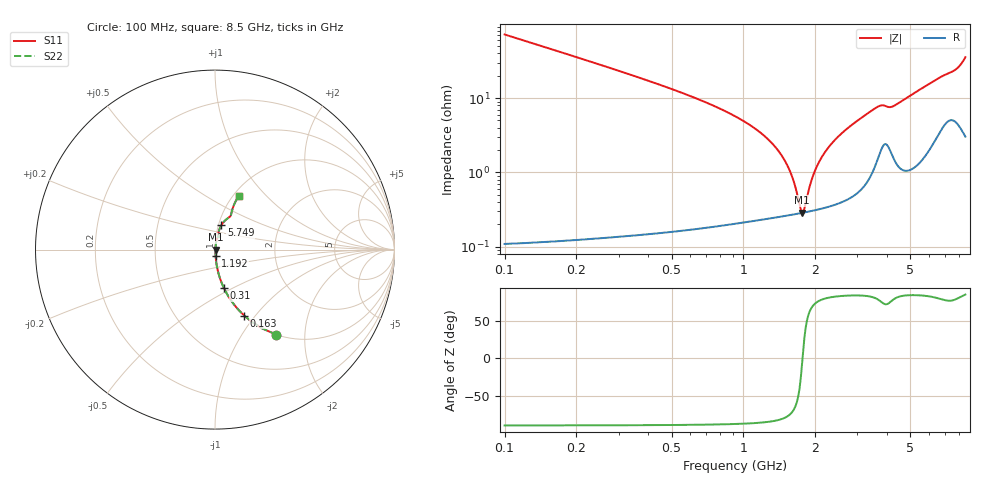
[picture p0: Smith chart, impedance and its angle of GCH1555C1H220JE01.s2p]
!Murata Part Number: GCH1555C1H220JE01
!These Parameters are Measured in Series Mode Connection
!Data Generated on Jun 19, 2026
!  o--ll--o
!Port1  Port2
!  o------o
!Operation Temp=25[degC], DC Bias Voltage=0[V]
!Freq. Start=100[MHz] Stop=9[GHz] 401[Steps]
# Hz S RI R 50
!Freq.(Hz) S11(Real) S11(Imag) S21(Real) S21(Imag) S12(Real) S12(Imag) S22(Real) S22(Imag)
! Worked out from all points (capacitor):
!   401 points, 100 MHz to 8.5 GHz, reference 50 ohm
!   read as one part in series: C = 22 pF near 142 MHz
!   lowest |Z| = 287 mohm at 1.759 GHz (marker M1)
!   series resonance near 1.768 GHz, so ESL is about 370 pH
!   S11 on the Smith chart (normalised r, x): 100 MHz: 1.00, -1.44; 163 MHz: 1.00, -0.88; 310 MHz: 1.00, -0.45; 1.192 GHz: 1.00, -0.07; 5.749 GHz: 1.03, +0.29; 8.5 GHz: 1.06, +0.71
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1e8  0.3422 -0.4737  0.6578 0.4737  0.6578 0.4737  0.3422 -0.4737
1.63e8  0.1628 -0.3678  0.8372 0.3678  0.8372 0.3678  0.1628 -0.3678
3.1e8  0.0497 -0.2144  0.9503 0.2144  0.9503 0.2144  0.0497 -0.2144
6.25e8  0.0118 -0.0998  0.9882 0.0998  0.9882 0.0998  0.0118 -0.0998
1.192e9  0.00339 -0.033  0.9966 0.033  0.9966 0.033  0.00339 -0.033
1.381e9  0.00289 -0.0204  0.9971 0.0204  0.9971 0.0204  0.00289 -0.0204
1.507e9  0.00277 -0.0132  0.9972 0.0132  0.9972 0.0132  0.00277 -0.0132
1.591e9  0.00275 -0.00869  0.9973 0.00869  0.9973 0.00869  0.00275 -0.00869
1.717e9  0.0028 -0.00242  0.9972 0.00242  0.9972 0.00242  0.0028 -0.00242
1.759e9  0.00283 -0.000423  0.9972 0.000423  0.9972 0.000423  0.00283 -0.000423
1.801e9  0.00288 0.00153  0.9971 -0.00153  0.9971 -0.00153  0.00288 0.00153
1.969e9  0.00313 0.00897  0.9969 -0.00897  0.9969 -0.00897  0.00313 0.00897
2.158e9  0.00356 0.0168  0.9964 -0.0168  0.9964 -0.0168  0.00356 0.0168
2.473e9  0.00459 0.029  0.9954 -0.029  0.9954 -0.029  0.00459 0.029
2.914e9  0.00695 0.0455  0.993 -0.0455  0.993 -0.0455  0.00695 0.0455
3.67e9  0.021 0.0729  0.979 -0.0729  0.979 -0.0729  0.021 0.0729
4.3e9  0.02 0.0757  0.98 -0.0757  0.98 -0.0757  0.02 0.0757
5.707e9  0.034 0.1336  0.966 -0.1336  0.966 -0.1336  0.034 0.1336
5.749e9  0.035 0.1353  0.965 -0.1353  0.965 -0.1353  0.035 0.1353
7.114e9  0.0808 0.1812  0.9192 -0.1812  0.9192 -0.1812  0.0808 0.1812
7.849e9  0.0944 0.215  0.9056 -0.215  0.9056 -0.215  0.0944 0.215
8.5e9  0.1326 0.2992  0.8674 -0.2992  0.8674 -0.2992  0.1326 0.2992
